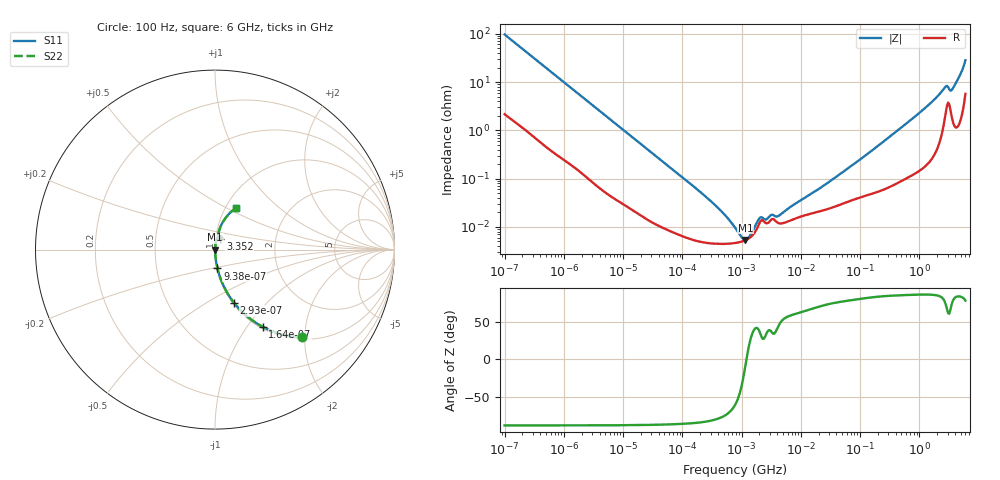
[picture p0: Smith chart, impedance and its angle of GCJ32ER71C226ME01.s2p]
!Murata Part Number: GCJ32ER71C226ME01
!These Parameters are Measured in Series Mode Connection
!Data Generated on Mar 13, 2026
!  o--ll--o
!Port1  Port2
!  o------o
!Operation Temp=25[degC], DC Bias Voltage=0[V]
!Freq. Start=100[Hz] Stop=6[GHz] 401[Steps]
# Hz S RI R 50
!Freq.(Hz) S11(Real) S11(Imag) S21(Real) S21(Imag) S12(Real) S12(Imag) S22(Real) S22(Imag)
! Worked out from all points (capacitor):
!   401 points, 100 Hz to 6 GHz, reference 50 ohm
!   read as one part in series: C = 16.4 uF near 109 Hz
!   lowest |Z| = 5.37 mohm at 1.159 MHz (marker M1)
!   series resonance near 1.211 MHz, so ESL is about 1.1 nH
!   S11 on the Smith chart (normalised r, x): 100 Hz: 1.04, -1.93; 164 Hz: 1.03, -1.19; 293 Hz: 1.02, -0.67; 938 Hz: 1.01, -0.21; 3.352 GHz: 1.05, +0.12; 6 GHz: 1.11, +0.55
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100  0.4838 -0.4887  0.5162 0.4887  0.5162 0.4887  0.4838 -0.4887
164  0.2663 -0.4307  0.7337 0.4307  0.7337 0.4307  0.2663 -0.4307
293  0.1067 -0.2974  0.8933 0.2974  0.8933 0.2974  0.1067 -0.2974
938  0.0137 -0.1047  0.9863 0.1047  0.9863 0.1047  0.0137 -0.1047
2008  0.00381 -0.0501  0.9962 0.0501  0.9962 0.0501  0.00381 -0.0501
40335  0.000111 -0.00262  0.9999 0.00262  0.9999 0.00262  0.000111 -0.00262
289253  4.6e-05 -0.000356  1 0.000356  1 0.000356  4.6e-05 -0.000356
774597  4.64e-05 -8.51e-05  1 8.51e-05  1 8.51e-05  4.64e-05 -8.51e-05
1159002  5.3e-05 -8.4e-06  0.9999 8.4e-06  0.9999 8.4e-06  5.3e-05 -8.4e-06
1585629  7.05e-05 5.45e-05  0.9999 -5.45e-05  0.9999 -5.45e-05  7.05e-05 5.45e-05
2074311  0.000131 8.85e-05  0.9999 -8.85e-05  0.9999 -8.85e-05  0.000131 8.85e-05
2594782  0.000119 7.83e-05  0.9999 -7.83e-05  0.9999 -7.83e-05  0.000119 7.83e-05
3245845  0.000145 0.000105  0.9999 -0.000105  0.9999 -0.000105  0.000145 0.000105
4246196  0.00012 0.000121  0.9999 -0.000121  0.9999 -0.000121  0.00012 0.000121
1.555665e7  0.000191 0.000459  0.9998 -0.000459  0.9998 -0.000459  0.000191 0.000459
3.124326e8  0.000719 0.00726  0.9993 -0.00726  0.9993 -0.00726  0.000719 0.00726
1.309207e9  0.00279 0.0302  0.9972 -0.0302  0.9972 -0.0302  0.00279 0.0302
2.679998e9  0.0219 0.0718  0.9781 -0.0718  0.9781 -0.0718  0.0219 0.0718
3.352442e9  0.0293 0.0573  0.9707 -0.0573  0.9707 -0.0573  0.0293 0.0573
3.8344e9  0.0189 0.077  0.9811 -0.077  0.9811 -0.077  0.0189 0.077
5.016141e9  0.0375 0.1418  0.9625 -0.1418  0.9625 -0.1418  0.0375 0.1418
6e9  0.1149 0.2321  0.8851 -0.2321  0.8851 -0.2321  0.1149 0.2321
